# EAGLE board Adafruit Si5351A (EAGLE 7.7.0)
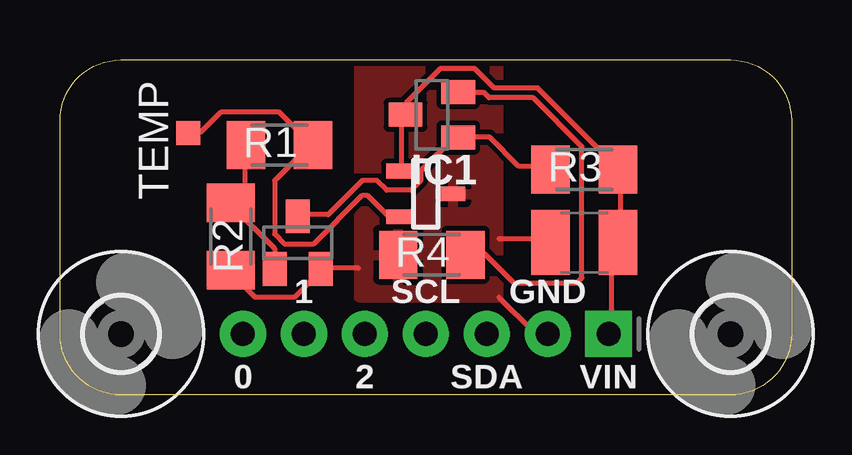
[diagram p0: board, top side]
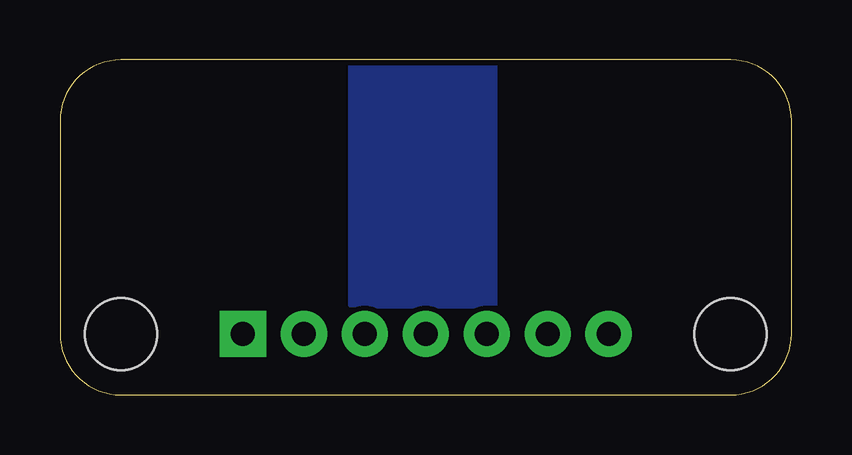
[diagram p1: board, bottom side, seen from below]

Size 30.48 x 13.97 mm. Coordinates in mm from the lower left corner, seen from the top.
Outline: 0,2.54 0,11.43 arc-90 2.54,13.97 27.94,13.97 arc-90 30.48,11.43 30.48,2.54 arc-90 27.94,0 2.54,0 arc-90 0,2.54
Copper layers (1*16): Top 0.035mm / dielectric 1.5mm / Bottom 0.035mm
Design rules "adafruit": minimum track width 8mil, minimum drill 15.5mil, track to track 8mil, track to pad 8mil, pad to pad 8mil, via to via 8mil, smd to smd 8mil, copper to edge 10mil, drill to drill 8mil, minimum pad ring 10mil, minimum via ring 8mil, stop-mask expansion 2mil, vias tented up to drill 20mil, thermal gap 10mil

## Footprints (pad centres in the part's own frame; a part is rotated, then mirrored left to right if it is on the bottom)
C1210 = smd 1.6 x 2.7: 1 -1.4,0; 2 1.4,0
3,0 = hole 3: 0,0
SOT23-3 = smd 0.61 x 1.016: 1 -0.953,-1.143; 2 0.953,-1.143; 3 0,1.143
1X07_ROUND_76 = drill 1 pad 1.93 square: 1 -7.62,0 | drill 1 pad 1.93: 2 -5.08,0; 3 -2.54,0; 4 0,0; 5 2.54,0; 6 5.08,0; 7 7.62,0
M1206 = smd 1.6 x 2: 1 -1.4,0; 2 1.4,0
SOT23 = smd 1 x 1.4: 1 -0.95,-1.1; 2 0.95,-1.1; 3 0,1.1
TP10SQ = smd 1 x 1: TP 0,0

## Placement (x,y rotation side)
C1  1uF  [C1210]  21.84,6.35 180 top
H1  MOUNT-HOLE3.0  [3,0]  27.94,2.54 0 top
H2  MOUNT-HOLE3.0  [3,0]  2.54,2.54 0 top
IC1  MCP9701 smd  [SOT23-3]  15.24,8.38 270 top
JP1  [1X07_ROUND_76]  15.24,2.54 180 top
R1  680  [M1206]  9.14,10.41 0 top
R2  680  [M1206]  7.11,6.6 90 top
R3  680  [M1206]  21.84,9.4 0 top
R4  2x22  [M1206]  15.49,5.84 0 top
T1  BC848  [SOT23]  9.91,6.35 0 top
T2  BC848  [SOT23]  15.49,11.68 90 top
TEMP  PTR1TP10SQ  [TP10SQ]  5.33,10.92 0 top

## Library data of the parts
C1 R1-R4 = rcl
H1 H2 = holes
IC1 = interGATE4
JP1 = microbuilder
T1 T2 = transistor
TEMP = testpad

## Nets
B1: R1.1 R2.2 T1.1
B2: R3.1 T1.3 T2.1
CLK0: JP1.7
CLK1: JP1.6
CLK2: JP1.5
E2: R4.2 T2.2
GND: C1.2 IC1.3 JP1.2 R2.1 R4.1 T1.2
SCL_5V: JP1.4
SDA_5V: JP1.3
TEMP: IC1.2 R1.2 TEMP.TP
VCC: C1.1 IC1.1 JP1.1 R3.2 T2.3

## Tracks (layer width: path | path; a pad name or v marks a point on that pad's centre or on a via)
B1
  Top 0.203: T1.1 8.94,5.28 8.94,6.1 7.11,7.92 R2.2 7.11,8.13 7.72,8.74 7.72,10.36 R1.1
B2
  Top 0.203: T1.3 9.96,7.52 11.18,7.52 12.6,8.94 13.21,8.94 13.61,8.53 14.63,8.53 15.04,8.94 15.04,9.35 16.46,10.77 T2.1 16.66,10.77 17.88,10.77 19.1,9.55 20.32,9.55 R3.1
E2
  Top 0.203: T2.2 16.66,12.6 17.68,12.6 17.88,12.39 19.71,12.39 21.74,10.36 21.74,4.88 21.54,4.67 18.9,4.67 17.68,5.89 17.07,5.89 R4.2
GND
  Top 0.203: 12.45,5.28 10.97,5.28 T1.2 10.77,5.08 9.75,4.06 8.13,4.06 7.11,5.08 R2.1 | 18.29,6.5 20.32,6.5 C1.2 | 18.29,4.06 19.71,2.64 20.32,2.64 JP1.2
  pour Top: 12.45,4.06 18.29,4.06 18.29,13.97 12.45,13.97
  pour Bottom: 12.45,13.72 18.29,13.72 18.29,3.81 12.45,3.81
TEMP
  Top 0.203: IC1.2 14.02,7.52 13.61,7.52 12.8,8.33 12.6,8.33 10.57,6.3 9.35,6.3 8.94,6.71 8.94,8.94 10.36,10.36 R1.2 10.36,10.57 9.14,11.79 6.71,11.79 5.89,10.97 5.49,10.97 TEMP.TP
VCC
  Top 0.203: IC1.1 14.22,9.35 14.22,11.58 T2.3 14.43,11.79 14.43,12.19 15.85,13.61 17.27,13.61 18.09,12.8 19.91,12.8 23.16,9.55 R3.2 23.37,9.35 23.37,6.5 C1.1 23.16,6.3 22.96,6.1 22.96,2.64 JP1.1

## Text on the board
tPlace: 1 | SCL | GND | 0 | 2 | SDA | VIN

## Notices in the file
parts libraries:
microbuilder: This work is placed in the public domain, and may be freely used for commercial and non-commercial work with the following conditions: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
